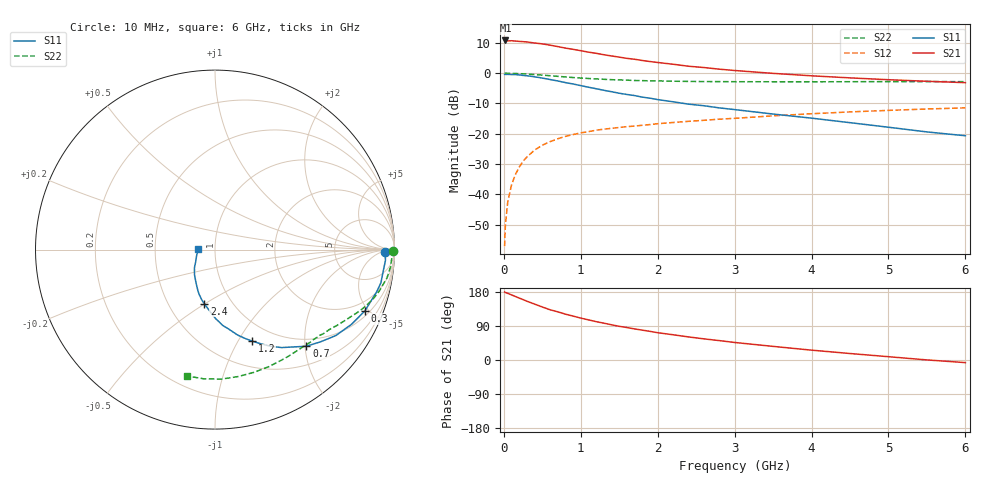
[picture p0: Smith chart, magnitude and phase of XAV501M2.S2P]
! SIEMENS Discrete & RF Semiconductors
! BFY180
! Si NPN RF Bipolar Junction Transistor in MICRO-X
! VCE = 0.5 V  IC = 1.2 mA
! Common Emitter S-Parameters:  May  1997
# GHz  S  MA  R  50
!  f  S11  S21  S12  S22
! GHz  MAG  ANG  MAG  ANG  MAG  ANG  MAG  ANG
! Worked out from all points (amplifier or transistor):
!   36 points, 10 MHz to 6 GHz, reference 50 ohm
!   highest |S21| = 10.7 dB at 20 MHz (marker M1)
!   |S21| within 3 dB of that: start of sweep to 917.5 MHz
!   unconditionally stable (mu >= 1): 1.631 GHz to end of sweep
!   at 250 MHz: K = 0.18, MSG = 19.7 dB, |S12| = -29.1 dB
!   at 1.4 GHz: K = 0.91, MSG = 11.9 dB, |S12| = -18.2 dB
!   at 6 GHz: K = 1.37, MAG = 0.5 dB, |S12| = -11.5 dB
!   S11 on the Smith chart (normalised r, x): 10 MHz: 36, -9; 300 MHz: 1.30, -4.76; 700 MHz: 0.85, -2.03; 1.2 GHz: 0.78, -1.15; 2.4 GHz: 0.75, -0.50; 6 GHz: 0.83, +0.01
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0.01  0.9488 -0.8  3.396 179.4  0.0014 92.1  0.9894 -0.4
0.02  0.948 -1.4  3.443 178.3  0.0031 89.0  0.9959 -0.8
0.05  0.9518 -3.6  3.386 176.0  0.0074 84.2  0.988 -1.9
0.1  0.9445 -7.5  3.407 171.8  0.0143 84.8  0.9844 -3.8
0.2  0.9312 -14.6  3.326 163.4  0.0281 80.1  0.9759 -7.5
0.3  0.9024 -22.2  3.258 155.1  0.0413 74.7  0.9613 -10.9
0.5  0.8263 -35.4  3.024 139.9  0.0646 65.6  0.9238 -17.2
0.6  0.7812 -41.1  2.882 132.6  0.0739 62.0  0.903 -19.7
0.7  0.7409 -46.6  2.73 127.2  0.0823 58.3  0.8825 -22.2
0.8  0.696 -51.2  2.576 121.0  0.0903 55.6  0.8618 -24.4
0.9  0.66 -55.8  2.46 115.9  0.0969 52.8  0.8431 -26.4
1.1  0.5831 -64.1  2.21 105.9  0.1082 48.6  0.8131 -30.1
1.2  0.5513 -67.8  2.114 101.2  0.1142 46.4  0.7999 -31.9
1.5  0.4645 -78.3  1.829 88.9  0.1267 42.1  0.7698 -36.6
1.7  0.4254 -84.1  1.687 82.0  0.1336 40.1  0.7533 -39.4
2.2  0.3359 -96.1  1.396 66.6  0.153 35.3  0.7333 -46.8
2.4  0.307 -101.3  1.295 60.9  0.1598 33.6  0.7274 -49.6
3  0.2497 -112.3  1.101 46.3  0.1792 29.0  0.7195 -58.0
3.5  0.2108 -120.3  0.987 35.9  0.197 25.6  0.7178 -65.2
4.5  0.152 -138.8  0.832 17.1  0.2286 16.7  0.719 -79.7
5.5  0.107 -162.7  0.731 0.2  0.2554 7.6  0.7228 -94.8
6  0.0925 177.6  0.694 -6.9  0.2666 2.9  0.7209 -102.3
